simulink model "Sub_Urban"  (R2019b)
settings: Solver=FixedStepAuto  StartTime=0.0  StopTime=3600*24  FixedStep=Tstep  MaxStep=1800  RelTol=1e-3
InitFcn:
  | load('network_parameters')
  | Vnom=400/sqrt(3);
  | Tstep=30*60;
  | MV_LV_transf=0;
StopFcn:
  | run('Simulink_Data.m')
undefined symbols (not defined in the file or in its folder): C_xlpe_185_90, D11, Delta, L_2x16mm, L_2x22mm, L_4x100mm, L_4x16mm, L_4x22mm, L_4x50mm, L_xlpe_185_90, LC, Line_length, R_2x16mm, R_2x22mm, R_4x100mm, R_4x16mm, R_4x22mm, R_4x50mm, R_xlpe_185_90, Source_Voltage
libraries: myLibrary x125, powerlib x89
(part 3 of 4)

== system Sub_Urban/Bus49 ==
  Three Phase Zero Bus : myLibrary/Three Phase Zero Bus  SystemSampleTime=-1  Latency=0  AutoFrameSizeCalculation=off
  To Workspace I : ToWorkspace  VariableName=I49  SaveFormat=Structure With Time  SampleTime=-1
  To Workspace V : ToWorkspace  VariableName=Bus49  SaveFormat=Structure With Time  SampleTime=-1
  A : PMIOPort  Tag=PMCPort  Side=Left
  B : PMIOPort  Tag=PMCPort  Port=2  Side=Left
  C : PMIOPort  Tag=PMCPort  Port=3  Side=Left
  N : PMIOPort  Tag=PMCPort  Port=4  Side=Left
  a : PMIOPort  Tag=PMCPort  Port=5  Side=Right
  b : PMIOPort  Tag=PMCPort  Port=6  Side=Right
  c : PMIOPort  Tag=PMCPort  Port=7  Side=Right
  n : PMIOPort  Tag=PMCPort  Port=8  Side=Right
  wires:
  Three Phase Zero Bus/1 -> To Workspace V/1
  Three Phase Zero Bus/2 -> To Workspace I/1
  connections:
  A/RConn1 -- Three Phase Zero Bus/LConn1
  B/RConn1 -- Three Phase Zero Bus/LConn2
  C/RConn1 -- Three Phase Zero Bus/LConn3
  N/RConn1 -- Three Phase Zero Bus/LConn4
  a/RConn1 -- Three Phase Zero Bus/RConn1
  b/RConn1 -- Three Phase Zero Bus/RConn2
  c/RConn1 -- Three Phase Zero Bus/RConn3
  n/RConn1 -- Three Phase Zero Bus/RConn4

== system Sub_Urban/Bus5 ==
  Three Phase Zero Bus : myLibrary/Three Phase Zero Bus  SystemSampleTime=-1  Latency=0  AutoFrameSizeCalculation=off
  To Workspace I : ToWorkspace  VariableName=I5  SaveFormat=Structure With Time  SampleTime=-1
  To Workspace V : ToWorkspace  VariableName=Bus5  SaveFormat=Structure With Time  SampleTime=-1
  A : PMIOPort  Tag=PMCPort  Side=Left
  B : PMIOPort  Tag=PMCPort  Port=2  Side=Left
  C : PMIOPort  Tag=PMCPort  Port=3  Side=Left
  N : PMIOPort  Tag=PMCPort  Port=4  Side=Left
  a : PMIOPort  Tag=PMCPort  Port=5  Side=Right
  b : PMIOPort  Tag=PMCPort  Port=6  Side=Right
  c : PMIOPort  Tag=PMCPort  Port=7  Side=Right
  n : PMIOPort  Tag=PMCPort  Port=8  Side=Right
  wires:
  Three Phase Zero Bus/1 -> To Workspace V/1
  Three Phase Zero Bus/2 -> To Workspace I/1
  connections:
  A/RConn1 -- Three Phase Zero Bus/LConn1
  B/RConn1 -- Three Phase Zero Bus/LConn2
  C/RConn1 -- Three Phase Zero Bus/LConn3
  N/RConn1 -- Three Phase Zero Bus/LConn4
  a/RConn1 -- Three Phase Zero Bus/RConn1
  b/RConn1 -- Three Phase Zero Bus/RConn2
  c/RConn1 -- Three Phase Zero Bus/RConn3
  n/RConn1 -- Three Phase Zero Bus/RConn4

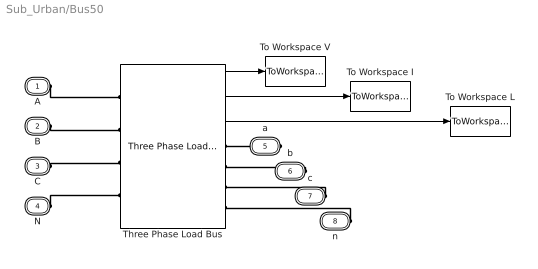
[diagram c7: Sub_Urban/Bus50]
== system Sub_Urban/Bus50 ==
  Three Phase Load Bus : myLibrary/Three Phase Load Bus  SystemSampleTime=-1  Latency=0  AutoFrameSizeCalculation=off
  To Workspace I : ToWorkspace  VariableName=I50  SaveFormat=Structure With Time  SampleTime=-1
  To Workspace L : ToWorkspace  VariableName=Load32  SaveFormat=Structure With Time  SampleTime=-1
  To Workspace V : ToWorkspace  VariableName=Bus50  SaveFormat=Structure With Time  SampleTime=-1
  A : PMIOPort  Tag=PMCPort  Side=Left
  B : PMIOPort  Tag=PMCPort  Port=2  Side=Left
  C : PMIOPort  Tag=PMCPort  Port=3  Side=Left
  N : PMIOPort  Tag=PMCPort  Port=4  Side=Left
  a : PMIOPort  Tag=PMCPort  Port=5  Side=Right
  b : PMIOPort  Tag=PMCPort  Port=6  Side=Right
  c : PMIOPort  Tag=PMCPort  Port=7  Side=Right
  n : PMIOPort  Tag=PMCPort  Port=8  Side=Right
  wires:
  Three Phase Load Bus/1 -> To Workspace V/1
  Three Phase Load Bus/2 -> To Workspace I/1
  Three Phase Load Bus/3 -> To Workspace L/1
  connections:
  N/RConn1 -- Three Phase Load Bus/LConn4
  C/RConn1 -- Three Phase Load Bus/LConn3
  n/RConn1 -- Three Phase Load Bus/RConn4
  B/RConn1 -- Three Phase Load Bus/LConn2
  A/RConn1 -- Three Phase Load Bus/LConn1
  b/RConn1 -- Three Phase Load Bus/RConn2
  c/RConn1 -- Three Phase Load Bus/RConn3
  a/RConn1 -- Three Phase Load Bus/RConn1

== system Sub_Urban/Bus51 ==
  Constant : Constant  Value=Ph
  Single Phase Load Bus : myLibrary/Single Phase Load Bus  SystemSampleTime=-1  Latency=0  AutoFrameSizeCalculation=off
  To Workspace I : ToWorkspace  VariableName=I51  SaveFormat=Structure With Time  SampleTime=-1
  To Workspace L : ToWorkspace  VariableName=Load33  SaveFormat=Structure With Time  SampleTime=-1
  To Workspace V : ToWorkspace  VariableName=Bus51  SaveFormat=Structure With Time  SampleTime=-1
  Phase : PMIOPort  Tag=PMCPort  Side=Left
  N : PMIOPort  Tag=PMCPort  Port=2  Side=Left
  phase : PMIOPort  Tag=PMCPort  Port=3  Side=Right
  n : PMIOPort  Tag=PMCPort  Port=4  Side=Right
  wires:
  Constant/1 -> Single Phase Load Bus/1
  Single Phase Load Bus/1 -> To Workspace V/1
  Single Phase Load Bus/2 -> To Workspace I/1
  Single Phase Load Bus/3 -> To Workspace L/1
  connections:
  Phase/RConn1 -- Single Phase Load Bus/LConn1
  N/RConn1 -- Single Phase Load Bus/LConn2
  phase/RConn1 -- Single Phase Load Bus/RConn1
  n/RConn1 -- Single Phase Load Bus/RConn2

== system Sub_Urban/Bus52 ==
  Three Phase Zero Bus : myLibrary/Three Phase Zero Bus  SystemSampleTime=-1  Latency=0  AutoFrameSizeCalculation=off
  To Workspace I : ToWorkspace  VariableName=I52  SaveFormat=Structure With Time  SampleTime=-1
  To Workspace V : ToWorkspace  VariableName=Bus52  SaveFormat=Structure With Time  SampleTime=-1
  A : PMIOPort  Tag=PMCPort  Side=Left
  B : PMIOPort  Tag=PMCPort  Port=2  Side=Left
  C : PMIOPort  Tag=PMCPort  Port=3  Side=Left
  N : PMIOPort  Tag=PMCPort  Port=4  Side=Left
  a : PMIOPort  Tag=PMCPort  Port=5  Side=Right
  b : PMIOPort  Tag=PMCPort  Port=6  Side=Right
  c : PMIOPort  Tag=PMCPort  Port=7  Side=Right
  n : PMIOPort  Tag=PMCPort  Port=8  Side=Right
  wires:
  Three Phase Zero Bus/1 -> To Workspace V/1
  Three Phase Zero Bus/2 -> To Workspace I/1
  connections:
  A/RConn1 -- Three Phase Zero Bus/LConn1
  B/RConn1 -- Three Phase Zero Bus/LConn2
  C/RConn1 -- Three Phase Zero Bus/LConn3
  N/RConn1 -- Three Phase Zero Bus/LConn4
  a/RConn1 -- Three Phase Zero Bus/RConn1
  b/RConn1 -- Three Phase Zero Bus/RConn2
  c/RConn1 -- Three Phase Zero Bus/RConn3
  n/RConn1 -- Three Phase Zero Bus/RConn4

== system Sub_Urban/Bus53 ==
  Constant : Constant  Value=Ph
  Single Phase Load Bus : myLibrary/Single Phase Load Bus  SystemSampleTime=-1  Latency=0  AutoFrameSizeCalculation=off
  To Workspace I : ToWorkspace  VariableName=I53  SaveFormat=Structure With Time  SampleTime=-1
  To Workspace L : ToWorkspace  VariableName=Load34  SaveFormat=Structure With Time  SampleTime=-1
  To Workspace V : ToWorkspace  VariableName=Bus53  SaveFormat=Structure With Time  SampleTime=-1
  Phase : PMIOPort  Tag=PMCPort  Side=Left
  N : PMIOPort  Tag=PMCPort  Port=2  Side=Left
  phase : PMIOPort  Tag=PMCPort  Port=3  Side=Right
  n : PMIOPort  Tag=PMCPort  Port=4  Side=Right
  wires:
  Constant/1 -> Single Phase Load Bus/1
  Single Phase Load Bus/1 -> To Workspace V/1
  Single Phase Load Bus/2 -> To Workspace I/1
  Single Phase Load Bus/3 -> To Workspace L/1
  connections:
  Phase/RConn1 -- Single Phase Load Bus/LConn1
  N/RConn1 -- Single Phase Load Bus/LConn2
  phase/RConn1 -- Single Phase Load Bus/RConn1
  n/RConn1 -- Single Phase Load Bus/RConn2

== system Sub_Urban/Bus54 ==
  Constant : Constant  Value=Ph
  Single Phase Load Bus : myLibrary/Single Phase Load Bus  SystemSampleTime=-1  Latency=0  AutoFrameSizeCalculation=off
  To Workspace I : ToWorkspace  VariableName=I54  SaveFormat=Structure With Time  SampleTime=-1
  To Workspace L : ToWorkspace  VariableName=Load35  SaveFormat=Structure With Time  SampleTime=-1
  To Workspace V : ToWorkspace  VariableName=Bus54  SaveFormat=Structure With Time  SampleTime=-1
  Phase : PMIOPort  Tag=PMCPort  Side=Left
  N : PMIOPort  Tag=PMCPort  Port=2  Side=Left
  phase : PMIOPort  Tag=PMCPort  Port=3  Side=Right
  n : PMIOPort  Tag=PMCPort  Port=4  Side=Right
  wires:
  Constant/1 -> Single Phase Load Bus/1
  Single Phase Load Bus/1 -> To Workspace V/1
  Single Phase Load Bus/2 -> To Workspace I/1
  Single Phase Load Bus/3 -> To Workspace L/1
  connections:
  Phase/RConn1 -- Single Phase Load Bus/LConn1
  N/RConn1 -- Single Phase Load Bus/LConn2
  phase/RConn1 -- Single Phase Load Bus/RConn1
  n/RConn1 -- Single Phase Load Bus/RConn2

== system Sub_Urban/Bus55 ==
  Three Phase Zero Bus : myLibrary/Three Phase Zero Bus  SystemSampleTime=-1  Latency=0  AutoFrameSizeCalculation=off
  To Workspace I : ToWorkspace  VariableName=I55  SaveFormat=Structure With Time  SampleTime=-1
  To Workspace V : ToWorkspace  VariableName=Bus55  SaveFormat=Structure With Time  SampleTime=-1
  A : PMIOPort  Tag=PMCPort  Side=Left
  B : PMIOPort  Tag=PMCPort  Port=2  Side=Left
  C : PMIOPort  Tag=PMCPort  Port=3  Side=Left
  N : PMIOPort  Tag=PMCPort  Port=4  Side=Left
  a : PMIOPort  Tag=PMCPort  Port=5  Side=Right
  b : PMIOPort  Tag=PMCPort  Port=6  Side=Right
  c : PMIOPort  Tag=PMCPort  Port=7  Side=Right
  n : PMIOPort  Tag=PMCPort  Port=8  Side=Right
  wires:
  Three Phase Zero Bus/1 -> To Workspace V/1
  Three Phase Zero Bus/2 -> To Workspace I/1
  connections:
  A/RConn1 -- Three Phase Zero Bus/LConn1
  B/RConn1 -- Three Phase Zero Bus/LConn2
  C/RConn1 -- Three Phase Zero Bus/LConn3
  N/RConn1 -- Three Phase Zero Bus/LConn4
  a/RConn1 -- Three Phase Zero Bus/RConn1
  b/RConn1 -- Three Phase Zero Bus/RConn2
  c/RConn1 -- Three Phase Zero Bus/RConn3
  n/RConn1 -- Three Phase Zero Bus/RConn4

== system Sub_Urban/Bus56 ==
  Constant : Constant  Value=Ph
  Single Phase Load Bus : myLibrary/Single Phase Load Bus  SystemSampleTime=-1  Latency=0  AutoFrameSizeCalculation=off
  To Workspace I : ToWorkspace  VariableName=I56  SaveFormat=Structure With Time  SampleTime=-1
  To Workspace L : ToWorkspace  VariableName=Load36  SaveFormat=Structure With Time  SampleTime=-1
  To Workspace V : ToWorkspace  VariableName=Bus56  SaveFormat=Structure With Time  SampleTime=-1
  Phase : PMIOPort  Tag=PMCPort  Side=Left
  N : PMIOPort  Tag=PMCPort  Port=2  Side=Left
  phase : PMIOPort  Tag=PMCPort  Port=3  Side=Right
  n : PMIOPort  Tag=PMCPort  Port=4  Side=Right
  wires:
  Constant/1 -> Single Phase Load Bus/1
  Single Phase Load Bus/1 -> To Workspace V/1
  Single Phase Load Bus/2 -> To Workspace I/1
  Single Phase Load Bus/3 -> To Workspace L/1
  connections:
  Phase/RConn1 -- Single Phase Load Bus/LConn1
  N/RConn1 -- Single Phase Load Bus/LConn2
  phase/RConn1 -- Single Phase Load Bus/RConn1
  n/RConn1 -- Single Phase Load Bus/RConn2

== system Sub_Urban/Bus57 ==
  Constant : Constant  Value=Ph
  Single Phase Load Bus : myLibrary/Single Phase Load Bus  SystemSampleTime=-1  Latency=0  AutoFrameSizeCalculation=off
  To Workspace I : ToWorkspace  VariableName=I57  SaveFormat=Structure With Time  SampleTime=-1
  To Workspace L : ToWorkspace  VariableName=Load37  SaveFormat=Structure With Time  SampleTime=-1
  To Workspace V : ToWorkspace  VariableName=Bus57  SaveFormat=Structure With Time  SampleTime=-1
  Phase : PMIOPort  Tag=PMCPort  Side=Left
  N : PMIOPort  Tag=PMCPort  Port=2  Side=Left
  phase : PMIOPort  Tag=PMCPort  Port=3  Side=Right
  n : PMIOPort  Tag=PMCPort  Port=4  Side=Right
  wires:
  Constant/1 -> Single Phase Load Bus/1
  Single Phase Load Bus/1 -> To Workspace V/1
  Single Phase Load Bus/2 -> To Workspace I/1
  Single Phase Load Bus/3 -> To Workspace L/1
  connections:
  Phase/RConn1 -- Single Phase Load Bus/LConn1
  N/RConn1 -- Single Phase Load Bus/LConn2
  phase/RConn1 -- Single Phase Load Bus/RConn1
  n/RConn1 -- Single Phase Load Bus/RConn2

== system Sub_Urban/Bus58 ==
  Three Phase Zero Bus : myLibrary/Three Phase Zero Bus  SystemSampleTime=-1  Latency=0  AutoFrameSizeCalculation=off
  To Workspace I : ToWorkspace  VariableName=I58  SaveFormat=Structure With Time  SampleTime=-1
  To Workspace V : ToWorkspace  VariableName=Bus58  SaveFormat=Structure With Time  SampleTime=-1
  A : PMIOPort  Tag=PMCPort  Side=Left
  B : PMIOPort  Tag=PMCPort  Port=2  Side=Left
  C : PMIOPort  Tag=PMCPort  Port=3  Side=Left
  N : PMIOPort  Tag=PMCPort  Port=4  Side=Left
  a : PMIOPort  Tag=PMCPort  Port=5  Side=Right
  b : PMIOPort  Tag=PMCPort  Port=6  Side=Right
  c : PMIOPort  Tag=PMCPort  Port=7  Side=Right
  n : PMIOPort  Tag=PMCPort  Port=8  Side=Right
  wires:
  Three Phase Zero Bus/1 -> To Workspace V/1
  Three Phase Zero Bus/2 -> To Workspace I/1
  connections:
  A/RConn1 -- Three Phase Zero Bus/LConn1
  B/RConn1 -- Three Phase Zero Bus/LConn2
  C/RConn1 -- Three Phase Zero Bus/LConn3
  N/RConn1 -- Three Phase Zero Bus/LConn4
  a/RConn1 -- Three Phase Zero Bus/RConn1
  b/RConn1 -- Three Phase Zero Bus/RConn2
  c/RConn1 -- Three Phase Zero Bus/RConn3
  n/RConn1 -- Three Phase Zero Bus/RConn4

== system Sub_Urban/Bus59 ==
  Constant : Constant  Value=Ph
  Single Phase Load Bus : myLibrary/Single Phase Load Bus  SystemSampleTime=-1  Latency=0  AutoFrameSizeCalculation=off
  To Workspace I : ToWorkspace  VariableName=I59  SaveFormat=Structure With Time  SampleTime=-1
  To Workspace L : ToWorkspace  VariableName=Load38  SaveFormat=Structure With Time  SampleTime=-1
  To Workspace V : ToWorkspace  VariableName=Bus59  SaveFormat=Structure With Time  SampleTime=-1
  Phase : PMIOPort  Tag=PMCPort  Side=Left
  N : PMIOPort  Tag=PMCPort  Port=2  Side=Left
  phase : PMIOPort  Tag=PMCPort  Port=3  Side=Right
  n : PMIOPort  Tag=PMCPort  Port=4  Side=Right
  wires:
  Constant/1 -> Single Phase Load Bus/1
  Single Phase Load Bus/1 -> To Workspace V/1
  Single Phase Load Bus/2 -> To Workspace I/1
  Single Phase Load Bus/3 -> To Workspace L/1
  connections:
  Phase/RConn1 -- Single Phase Load Bus/LConn1
  N/RConn1 -- Single Phase Load Bus/LConn2
  phase/RConn1 -- Single Phase Load Bus/RConn1
  n/RConn1 -- Single Phase Load Bus/RConn2

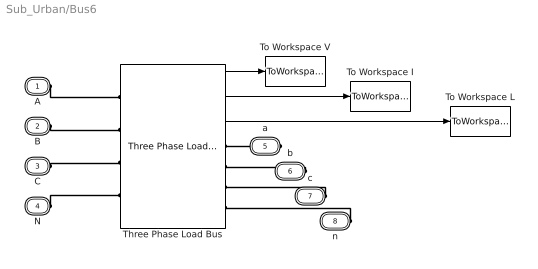
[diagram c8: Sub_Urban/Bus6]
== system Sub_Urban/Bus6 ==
  Three Phase Load Bus : myLibrary/Three Phase Load Bus  SystemSampleTime=-1  Latency=0  AutoFrameSizeCalculation=off
  To Workspace I : ToWorkspace  VariableName=I6  SaveFormat=Structure With Time  SampleTime=-1
  To Workspace L : ToWorkspace  VariableName=Load2  SaveFormat=Structure With Time  SampleTime=-1
  To Workspace V : ToWorkspace  VariableName=Bus6  SaveFormat=Structure With Time  SampleTime=-1
  A : PMIOPort  Tag=PMCPort  Side=Left
  B : PMIOPort  Tag=PMCPort  Port=2  Side=Left
  C : PMIOPort  Tag=PMCPort  Port=3  Side=Left
  N : PMIOPort  Tag=PMCPort  Port=4  Side=Left
  a : PMIOPort  Tag=PMCPort  Port=5  Side=Right
  b : PMIOPort  Tag=PMCPort  Port=6  Side=Right
  c : PMIOPort  Tag=PMCPort  Port=7  Side=Right
  n : PMIOPort  Tag=PMCPort  Port=8  Side=Right
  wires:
  Three Phase Load Bus/1 -> To Workspace V/1
  Three Phase Load Bus/2 -> To Workspace I/1
  Three Phase Load Bus/3 -> To Workspace L/1
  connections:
  N/RConn1 -- Three Phase Load Bus/LConn4
  C/RConn1 -- Three Phase Load Bus/LConn3
  n/RConn1 -- Three Phase Load Bus/RConn4
  B/RConn1 -- Three Phase Load Bus/LConn2
  A/RConn1 -- Three Phase Load Bus/LConn1
  b/RConn1 -- Three Phase Load Bus/RConn2
  c/RConn1 -- Three Phase Load Bus/RConn3
  a/RConn1 -- Three Phase Load Bus/RConn1

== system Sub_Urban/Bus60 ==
  Constant : Constant  Value=Ph
  Single Phase Load Bus : myLibrary/Single Phase Load Bus  SystemSampleTime=-1  Latency=0  AutoFrameSizeCalculation=off
  To Workspace I : ToWorkspace  VariableName=I60  SaveFormat=Structure With Time  SampleTime=-1
  To Workspace L : ToWorkspace  VariableName=Load39  SaveFormat=Structure With Time  SampleTime=-1
  To Workspace V : ToWorkspace  VariableName=Bus60  SaveFormat=Structure With Time  SampleTime=-1
  Phase : PMIOPort  Tag=PMCPort  Side=Left
  N : PMIOPort  Tag=PMCPort  Port=2  Side=Left
  phase : PMIOPort  Tag=PMCPort  Port=3  Side=Right
  n : PMIOPort  Tag=PMCPort  Port=4  Side=Right
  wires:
  Constant/1 -> Single Phase Load Bus/1
  Single Phase Load Bus/1 -> To Workspace V/1
  Single Phase Load Bus/2 -> To Workspace I/1
  Single Phase Load Bus/3 -> To Workspace L/1
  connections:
  Phase/RConn1 -- Single Phase Load Bus/LConn1
  N/RConn1 -- Single Phase Load Bus/LConn2
  phase/RConn1 -- Single Phase Load Bus/RConn1
  n/RConn1 -- Single Phase Load Bus/RConn2

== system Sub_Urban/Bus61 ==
  Constant : Constant  Value=Ph
  Single Phase Load Bus : myLibrary/Single Phase Load Bus  SystemSampleTime=-1  Latency=0  AutoFrameSizeCalculation=off
  To Workspace I : ToWorkspace  VariableName=I61  SaveFormat=Structure With Time  SampleTime=-1
  To Workspace L : ToWorkspace  VariableName=Load40  SaveFormat=Structure With Time  SampleTime=-1
  To Workspace V : ToWorkspace  VariableName=Bus61  SaveFormat=Structure With Time  SampleTime=-1
  Phase : PMIOPort  Tag=PMCPort  Side=Left
  N : PMIOPort  Tag=PMCPort  Port=2  Side=Left
  phase : PMIOPort  Tag=PMCPort  Port=3  Side=Right
  n : PMIOPort  Tag=PMCPort  Port=4  Side=Right
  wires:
  Constant/1 -> Single Phase Load Bus/1
  Single Phase Load Bus/1 -> To Workspace V/1
  Single Phase Load Bus/2 -> To Workspace I/1
  Single Phase Load Bus/3 -> To Workspace L/1
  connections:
  Phase/RConn1 -- Single Phase Load Bus/LConn1
  N/RConn1 -- Single Phase Load Bus/LConn2
  phase/RConn1 -- Single Phase Load Bus/RConn1
  n/RConn1 -- Single Phase Load Bus/RConn2

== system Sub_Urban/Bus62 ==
  Three Phase Zero Bus : myLibrary/Three Phase Zero Bus  SystemSampleTime=-1  Latency=0  AutoFrameSizeCalculation=off
  To Workspace I : ToWorkspace  VariableName=I62  SaveFormat=Structure With Time  SampleTime=-1
  To Workspace V : ToWorkspace  VariableName=Bus62  SaveFormat=Structure With Time  SampleTime=-1
  A : PMIOPort  Tag=PMCPort  Side=Left
  B : PMIOPort  Tag=PMCPort  Port=2  Side=Left
  C : PMIOPort  Tag=PMCPort  Port=3  Side=Left
  N : PMIOPort  Tag=PMCPort  Port=4  Side=Left
  a : PMIOPort  Tag=PMCPort  Port=5  Side=Right
  b : PMIOPort  Tag=PMCPort  Port=6  Side=Right
  c : PMIOPort  Tag=PMCPort  Port=7  Side=Right
  n : PMIOPort  Tag=PMCPort  Port=8  Side=Right
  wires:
  Three Phase Zero Bus/1 -> To Workspace V/1
  Three Phase Zero Bus/2 -> To Workspace I/1
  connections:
  A/RConn1 -- Three Phase Zero Bus/LConn1
  B/RConn1 -- Three Phase Zero Bus/LConn2
  C/RConn1 -- Three Phase Zero Bus/LConn3
  N/RConn1 -- Three Phase Zero Bus/LConn4
  a/RConn1 -- Three Phase Zero Bus/RConn1
  b/RConn1 -- Three Phase Zero Bus/RConn2
  c/RConn1 -- Three Phase Zero Bus/RConn3
  n/RConn1 -- Three Phase Zero Bus/RConn4

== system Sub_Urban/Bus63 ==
  Three Phase Zero Bus : myLibrary/Three Phase Zero Bus  SystemSampleTime=-1  Latency=0  AutoFrameSizeCalculation=off
  To Workspace I : ToWorkspace  VariableName=I63  SaveFormat=Structure With Time  SampleTime=-1
  To Workspace V : ToWorkspace  VariableName=Bus63  SaveFormat=Structure With Time  SampleTime=-1
  A : PMIOPort  Tag=PMCPort  Side=Left
  B : PMIOPort  Tag=PMCPort  Port=2  Side=Left
  C : PMIOPort  Tag=PMCPort  Port=3  Side=Left
  N : PMIOPort  Tag=PMCPort  Port=4  Side=Left
  a : PMIOPort  Tag=PMCPort  Port=5  Side=Right
  b : PMIOPort  Tag=PMCPort  Port=6  Side=Right
  c : PMIOPort  Tag=PMCPort  Port=7  Side=Right
  n : PMIOPort  Tag=PMCPort  Port=8  Side=Right
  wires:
  Three Phase Zero Bus/1 -> To Workspace V/1
  Three Phase Zero Bus/2 -> To Workspace I/1
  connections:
  A/RConn1 -- Three Phase Zero Bus/LConn1
  B/RConn1 -- Three Phase Zero Bus/LConn2
  C/RConn1 -- Three Phase Zero Bus/LConn3
  N/RConn1 -- Three Phase Zero Bus/LConn4
  a/RConn1 -- Three Phase Zero Bus/RConn1
  b/RConn1 -- Three Phase Zero Bus/RConn2
  c/RConn1 -- Three Phase Zero Bus/RConn3
  n/RConn1 -- Three Phase Zero Bus/RConn4

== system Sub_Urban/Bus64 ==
  Three Phase Load Bus : myLibrary/Three Phase Load Bus  SystemSampleTime=-1  Latency=0  AutoFrameSizeCalculation=off
  To Workspace I : ToWorkspace  VariableName=I64  SaveFormat=Structure With Time  SampleTime=-1
  To Workspace L : ToWorkspace  VariableName=Load41  SaveFormat=Structure With Time  SampleTime=-1
  To Workspace V : ToWorkspace  VariableName=Bus64  SaveFormat=Structure With Time  SampleTime=-1
  A : PMIOPort  Tag=PMCPort  Side=Left
  B : PMIOPort  Tag=PMCPort  Port=2  Side=Left
  C : PMIOPort  Tag=PMCPort  Port=3  Side=Left
  N : PMIOPort  Tag=PMCPort  Port=4  Side=Left
  a : PMIOPort  Tag=PMCPort  Port=5  Side=Right
  b : PMIOPort  Tag=PMCPort  Port=6  Side=Right
  c : PMIOPort  Tag=PMCPort  Port=7  Side=Right
  n : PMIOPort  Tag=PMCPort  Port=8  Side=Right
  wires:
  Three Phase Load Bus/1 -> To Workspace V/1
  Three Phase Load Bus/2 -> To Workspace I/1
  Three Phase Load Bus/3 -> To Workspace L/1
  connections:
  N/RConn1 -- Three Phase Load Bus/LConn4
  C/RConn1 -- Three Phase Load Bus/LConn3
  n/RConn1 -- Three Phase Load Bus/RConn4
  B/RConn1 -- Three Phase Load Bus/LConn2
  A/RConn1 -- Three Phase Load Bus/LConn1
  b/RConn1 -- Three Phase Load Bus/RConn2
  c/RConn1 -- Three Phase Load Bus/RConn3
  a/RConn1 -- Three Phase Load Bus/RConn1

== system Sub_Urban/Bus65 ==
  Constant : Constant  Value=Ph
  Single Phase Load Bus : myLibrary/Single Phase Load Bus  SystemSampleTime=-1  Latency=0  AutoFrameSizeCalculation=off
  To Workspace I : ToWorkspace  VariableName=I65  SaveFormat=Structure With Time  SampleTime=-1
  To Workspace L : ToWorkspace  VariableName=Load42  SaveFormat=Structure With Time  SampleTime=-1
  To Workspace V : ToWorkspace  VariableName=Bus65  SaveFormat=Structure With Time  SampleTime=-1
  Phase : PMIOPort  Tag=PMCPort  Side=Left
  N : PMIOPort  Tag=PMCPort  Port=2  Side=Left
  phase : PMIOPort  Tag=PMCPort  Port=3  Side=Right
  n : PMIOPort  Tag=PMCPort  Port=4  Side=Right
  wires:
  Constant/1 -> Single Phase Load Bus/1
  Single Phase Load Bus/1 -> To Workspace V/1
  Single Phase Load Bus/2 -> To Workspace I/1
  Single Phase Load Bus/3 -> To Workspace L/1
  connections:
  Phase/RConn1 -- Single Phase Load Bus/LConn1
  N/RConn1 -- Single Phase Load Bus/LConn2
  phase/RConn1 -- Single Phase Load Bus/RConn1
  n/RConn1 -- Single Phase Load Bus/RConn2

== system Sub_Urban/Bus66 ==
  Three Phase Zero Bus : myLibrary/Three Phase Zero Bus  SystemSampleTime=-1  Latency=0  AutoFrameSizeCalculation=off
  To Workspace I : ToWorkspace  VariableName=I66  SaveFormat=Structure With Time  SampleTime=-1
  To Workspace V : ToWorkspace  VariableName=Bus66  SaveFormat=Structure With Time  SampleTime=-1
  A : PMIOPort  Tag=PMCPort  Side=Left
  B : PMIOPort  Tag=PMCPort  Port=2  Side=Left
  C : PMIOPort  Tag=PMCPort  Port=3  Side=Left
  N : PMIOPort  Tag=PMCPort  Port=4  Side=Left
  a : PMIOPort  Tag=PMCPort  Port=5  Side=Right
  b : PMIOPort  Tag=PMCPort  Port=6  Side=Right
  c : PMIOPort  Tag=PMCPort  Port=7  Side=Right
  n : PMIOPort  Tag=PMCPort  Port=8  Side=Right
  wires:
  Three Phase Zero Bus/1 -> To Workspace V/1
  Three Phase Zero Bus/2 -> To Workspace I/1
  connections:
  A/RConn1 -- Three Phase Zero Bus/LConn1
  B/RConn1 -- Three Phase Zero Bus/LConn2
  C/RConn1 -- Three Phase Zero Bus/LConn3
  N/RConn1 -- Three Phase Zero Bus/LConn4
  a/RConn1 -- Three Phase Zero Bus/RConn1
  b/RConn1 -- Three Phase Zero Bus/RConn2
  c/RConn1 -- Three Phase Zero Bus/RConn3
  n/RConn1 -- Three Phase Zero Bus/RConn4

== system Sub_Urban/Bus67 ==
  Constant : Constant  Value=Ph
  Single Phase Load Bus : myLibrary/Single Phase Load Bus  SystemSampleTime=-1  Latency=0  AutoFrameSizeCalculation=off
  To Workspace I : ToWorkspace  VariableName=I67  SaveFormat=Structure With Time  SampleTime=-1
  To Workspace L : ToWorkspace  VariableName=Load43  SaveFormat=Structure With Time  SampleTime=-1
  To Workspace V : ToWorkspace  VariableName=Bus67  SaveFormat=Structure With Time  SampleTime=-1
  Phase : PMIOPort  Tag=PMCPort  Side=Left
  N : PMIOPort  Tag=PMCPort  Port=2  Side=Left
  phase : PMIOPort  Tag=PMCPort  Port=3  Side=Right
  n : PMIOPort  Tag=PMCPort  Port=4  Side=Right
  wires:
  Constant/1 -> Single Phase Load Bus/1
  Single Phase Load Bus/1 -> To Workspace V/1
  Single Phase Load Bus/2 -> To Workspace I/1
  Single Phase Load Bus/3 -> To Workspace L/1
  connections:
  Phase/RConn1 -- Single Phase Load Bus/LConn1
  N/RConn1 -- Single Phase Load Bus/LConn2
  phase/RConn1 -- Single Phase Load Bus/RConn1
  n/RConn1 -- Single Phase Load Bus/RConn2

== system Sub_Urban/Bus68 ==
  Constant : Constant  Value=Ph
  Single Phase Load Bus : myLibrary/Single Phase Load Bus  SystemSampleTime=-1  Latency=0  AutoFrameSizeCalculation=off
  To Workspace I : ToWorkspace  VariableName=I68  SaveFormat=Structure With Time  SampleTime=-1
  To Workspace L : ToWorkspace  VariableName=Load44  SaveFormat=Structure With Time  SampleTime=-1
  To Workspace V : ToWorkspace  VariableName=Bus68  SaveFormat=Structure With Time  SampleTime=-1
  Phase : PMIOPort  Tag=PMCPort  Side=Left
  N : PMIOPort  Tag=PMCPort  Port=2  Side=Left
  phase : PMIOPort  Tag=PMCPort  Port=3  Side=Right
  n : PMIOPort  Tag=PMCPort  Port=4  Side=Right
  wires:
  Constant/1 -> Single Phase Load Bus/1
  Single Phase Load Bus/1 -> To Workspace V/1
  Single Phase Load Bus/2 -> To Workspace I/1
  Single Phase Load Bus/3 -> To Workspace L/1
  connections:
  Phase/RConn1 -- Single Phase Load Bus/LConn1
  N/RConn1 -- Single Phase Load Bus/LConn2
  phase/RConn1 -- Single Phase Load Bus/RConn1
  n/RConn1 -- Single Phase Load Bus/RConn2

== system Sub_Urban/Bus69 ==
  Constant : Constant  Value=Ph
  Single Phase Load Bus : myLibrary/Single Phase Load Bus  SystemSampleTime=-1  Latency=0  AutoFrameSizeCalculation=off
  To Workspace I : ToWorkspace  VariableName=I69  SaveFormat=Structure With Time  SampleTime=-1
  To Workspace L : ToWorkspace  VariableName=Load45  SaveFormat=Structure With Time  SampleTime=-1
  To Workspace V : ToWorkspace  VariableName=Bus69  SaveFormat=Structure With Time  SampleTime=-1
  Phase : PMIOPort  Tag=PMCPort  Side=Left
  N : PMIOPort  Tag=PMCPort  Port=2  Side=Left
  phase : PMIOPort  Tag=PMCPort  Port=3  Side=Right
  n : PMIOPort  Tag=PMCPort  Port=4  Side=Right
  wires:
  Constant/1 -> Single Phase Load Bus/1
  Single Phase Load Bus/1 -> To Workspace V/1
  Single Phase Load Bus/2 -> To Workspace I/1
  Single Phase Load Bus/3 -> To Workspace L/1
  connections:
  Phase/RConn1 -- Single Phase Load Bus/LConn1
  N/RConn1 -- Single Phase Load Bus/LConn2
  phase/RConn1 -- Single Phase Load Bus/RConn1
  n/RConn1 -- Single Phase Load Bus/RConn2

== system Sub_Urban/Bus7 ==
  Constant : Constant  Value=Ph
  Single Phase Load Bus : myLibrary/Single Phase Load Bus  SystemSampleTime=-1  Latency=0  AutoFrameSizeCalculation=off
  To Workspace I : ToWorkspace  VariableName=I7  SaveFormat=Structure With Time  SampleTime=-1
  To Workspace L : ToWorkspace  VariableName=Load3  SaveFormat=Structure With Time  SampleTime=-1
  To Workspace V : ToWorkspace  VariableName=Bus7  SaveFormat=Structure With Time  SampleTime=-1
  Phase : PMIOPort  Tag=PMCPort  Side=Left
  N : PMIOPort  Tag=PMCPort  Port=2  Side=Left
  phase : PMIOPort  Tag=PMCPort  Port=3  Side=Right
  n : PMIOPort  Tag=PMCPort  Port=4  Side=Right
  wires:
  Constant/1 -> Single Phase Load Bus/1
  Single Phase Load Bus/1 -> To Workspace V/1
  Single Phase Load Bus/2 -> To Workspace I/1
  Single Phase Load Bus/3 -> To Workspace L/1
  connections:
  Phase/RConn1 -- Single Phase Load Bus/LConn1
  N/RConn1 -- Single Phase Load Bus/LConn2
  phase/RConn1 -- Single Phase Load Bus/RConn1
  n/RConn1 -- Single Phase Load Bus/RConn2

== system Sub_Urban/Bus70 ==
  Three Phase Zero Bus : myLibrary/Three Phase Zero Bus  SystemSampleTime=-1  Latency=0  AutoFrameSizeCalculation=off
  To Workspace I : ToWorkspace  VariableName=I70  SaveFormat=Structure With Time  SampleTime=-1
  To Workspace V : ToWorkspace  VariableName=Bus70  SaveFormat=Structure With Time  SampleTime=-1
  A : PMIOPort  Tag=PMCPort  Side=Left
  B : PMIOPort  Tag=PMCPort  Port=2  Side=Left
  C : PMIOPort  Tag=PMCPort  Port=3  Side=Left
  N : PMIOPort  Tag=PMCPort  Port=4  Side=Left
  a : PMIOPort  Tag=PMCPort  Port=5  Side=Right
  b : PMIOPort  Tag=PMCPort  Port=6  Side=Right
  c : PMIOPort  Tag=PMCPort  Port=7  Side=Right
  n : PMIOPort  Tag=PMCPort  Port=8  Side=Right
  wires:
  Three Phase Zero Bus/1 -> To Workspace V/1
  Three Phase Zero Bus/2 -> To Workspace I/1
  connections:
  A/RConn1 -- Three Phase Zero Bus/LConn1
  B/RConn1 -- Three Phase Zero Bus/LConn2
  C/RConn1 -- Three Phase Zero Bus/LConn3
  N/RConn1 -- Three Phase Zero Bus/LConn4
  a/RConn1 -- Three Phase Zero Bus/RConn1
  b/RConn1 -- Three Phase Zero Bus/RConn2
  c/RConn1 -- Three Phase Zero Bus/RConn3
  n/RConn1 -- Three Phase Zero Bus/RConn4

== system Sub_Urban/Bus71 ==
  Constant : Constant  Value=Ph
  Single Phase Load Bus : myLibrary/Single Phase Load Bus  SystemSampleTime=-1  Latency=0  AutoFrameSizeCalculation=off
  To Workspace I : ToWorkspace  VariableName=I71  SaveFormat=Structure With Time  SampleTime=-1
  To Workspace L : ToWorkspace  VariableName=Load46  SaveFormat=Structure With Time  SampleTime=-1
  To Workspace V : ToWorkspace  VariableName=Bus71  SaveFormat=Structure With Time  SampleTime=-1
  Phase : PMIOPort  Tag=PMCPort  Side=Left
  N : PMIOPort  Tag=PMCPort  Port=2  Side=Left
  phase : PMIOPort  Tag=PMCPort  Port=3  Side=Right
  n : PMIOPort  Tag=PMCPort  Port=4  Side=Right
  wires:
  Constant/1 -> Single Phase Load Bus/1
  Single Phase Load Bus/1 -> To Workspace V/1
  Single Phase Load Bus/2 -> To Workspace I/1
  Single Phase Load Bus/3 -> To Workspace L/1
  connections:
  Phase/RConn1 -- Single Phase Load Bus/LConn1
  N/RConn1 -- Single Phase Load Bus/LConn2
  phase/RConn1 -- Single Phase Load Bus/RConn1
  n/RConn1 -- Single Phase Load Bus/RConn2

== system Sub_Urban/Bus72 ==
  Constant : Constant  Value=Ph
  Single Phase Load Bus : myLibrary/Single Phase Load Bus  SystemSampleTime=-1  Latency=0  AutoFrameSizeCalculation=off
  To Workspace I : ToWorkspace  VariableName=I72  SaveFormat=Structure With Time  SampleTime=-1
  To Workspace L : ToWorkspace  VariableName=Load47  SaveFormat=Structure With Time  SampleTime=-1
  To Workspace V : ToWorkspace  VariableName=Bus72  SaveFormat=Structure With Time  SampleTime=-1
  Phase : PMIOPort  Tag=PMCPort  Side=Left
  N : PMIOPort  Tag=PMCPort  Port=2  Side=Left
  phase : PMIOPort  Tag=PMCPort  Port=3  Side=Right
  n : PMIOPort  Tag=PMCPort  Port=4  Side=Right
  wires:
  Constant/1 -> Single Phase Load Bus/1
  Single Phase Load Bus/1 -> To Workspace V/1
  Single Phase Load Bus/2 -> To Workspace I/1
  Single Phase Load Bus/3 -> To Workspace L/1
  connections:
  Phase/RConn1 -- Single Phase Load Bus/LConn1
  N/RConn1 -- Single Phase Load Bus/LConn2
  phase/RConn1 -- Single Phase Load Bus/RConn1
  n/RConn1 -- Single Phase Load Bus/RConn2

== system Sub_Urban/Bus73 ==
  Constant : Constant  Value=Ph
  Single Phase Load Bus : myLibrary/Single Phase Load Bus  SystemSampleTime=-1  Latency=0  AutoFrameSizeCalculation=off
  To Workspace I : ToWorkspace  VariableName=I73  SaveFormat=Structure With Time  SampleTime=-1
  To Workspace L : ToWorkspace  VariableName=Load48  SaveFormat=Structure With Time  SampleTime=-1
  To Workspace V : ToWorkspace  VariableName=Bus73  SaveFormat=Structure With Time  SampleTime=-1
  Phase : PMIOPort  Tag=PMCPort  Side=Left
  N : PMIOPort  Tag=PMCPort  Port=2  Side=Left
  phase : PMIOPort  Tag=PMCPort  Port=3  Side=Right
  n : PMIOPort  Tag=PMCPort  Port=4  Side=Right
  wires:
  Constant/1 -> Single Phase Load Bus/1
  Single Phase Load Bus/1 -> To Workspace V/1
  Single Phase Load Bus/2 -> To Workspace I/1
  Single Phase Load Bus/3 -> To Workspace L/1
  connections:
  Phase/RConn1 -- Single Phase Load Bus/LConn1
  N/RConn1 -- Single Phase Load Bus/LConn2
  phase/RConn1 -- Single Phase Load Bus/RConn1
  n/RConn1 -- Single Phase Load Bus/RConn2

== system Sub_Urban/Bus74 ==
  Three Phase Load Bus : myLibrary/Three Phase Load Bus  SystemSampleTime=-1  Latency=0  AutoFrameSizeCalculation=off
  To Workspace I : ToWorkspace  VariableName=I74  SaveFormat=Structure With Time  SampleTime=-1
  To Workspace L : ToWorkspace  VariableName=Load49  SaveFormat=Structure With Time  SampleTime=-1
  To Workspace V : ToWorkspace  VariableName=Bus74  SaveFormat=Structure With Time  SampleTime=-1
  A : PMIOPort  Tag=PMCPort  Side=Left
  B : PMIOPort  Tag=PMCPort  Port=2  Side=Left
  C : PMIOPort  Tag=PMCPort  Port=3  Side=Left
  N : PMIOPort  Tag=PMCPort  Port=4  Side=Left
  a : PMIOPort  Tag=PMCPort  Port=5  Side=Right
  b : PMIOPort  Tag=PMCPort  Port=6  Side=Right
  c : PMIOPort  Tag=PMCPort  Port=7  Side=Right
  n : PMIOPort  Tag=PMCPort  Port=8  Side=Right
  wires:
  Three Phase Load Bus/1 -> To Workspace V/1
  Three Phase Load Bus/2 -> To Workspace I/1
  Three Phase Load Bus/3 -> To Workspace L/1
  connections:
  N/RConn1 -- Three Phase Load Bus/LConn4
  C/RConn1 -- Three Phase Load Bus/LConn3
  n/RConn1 -- Three Phase Load Bus/RConn4
  B/RConn1 -- Three Phase Load Bus/LConn2
  A/RConn1 -- Three Phase Load Bus/LConn1
  b/RConn1 -- Three Phase Load Bus/RConn2
  c/RConn1 -- Three Phase Load Bus/RConn3
  a/RConn1 -- Three Phase Load Bus/RConn1

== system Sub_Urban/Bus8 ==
  Constant : Constant  Value=Ph
  Single Phase Load Bus : myLibrary/Single Phase Load Bus  SystemSampleTime=-1  Latency=0  AutoFrameSizeCalculation=off
  To Workspace I : ToWorkspace  VariableName=I8  SaveFormat=Structure With Time  SampleTime=-1
  To Workspace L : ToWorkspace  VariableName=Load4  SaveFormat=Structure With Time  SampleTime=-1
  To Workspace V : ToWorkspace  VariableName=Bus8  SaveFormat=Structure With Time  SampleTime=-1
  Phase : PMIOPort  Tag=PMCPort  Side=Left
  N : PMIOPort  Tag=PMCPort  Port=2  Side=Left
  phase : PMIOPort  Tag=PMCPort  Port=3  Side=Right
  n : PMIOPort  Tag=PMCPort  Port=4  Side=Right
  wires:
  Constant/1 -> Single Phase Load Bus/1
  Single Phase Load Bus/1 -> To Workspace V/1
  Single Phase Load Bus/2 -> To Workspace I/1
  Single Phase Load Bus/3 -> To Workspace L/1
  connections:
  Phase/RConn1 -- Single Phase Load Bus/LConn1
  N/RConn1 -- Single Phase Load Bus/LConn2
  phase/RConn1 -- Single Phase Load Bus/RConn1
  n/RConn1 -- Single Phase Load Bus/RConn2

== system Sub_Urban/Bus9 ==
  Three Phase Zero Bus : myLibrary/Three Phase Zero Bus  SystemSampleTime=-1  Latency=0  AutoFrameSizeCalculation=off
  To Workspace I : ToWorkspace  VariableName=I9  SaveFormat=Structure With Time  SampleTime=-1
  To Workspace V : ToWorkspace  VariableName=Bus9  SaveFormat=Structure With Time  SampleTime=-1
  A : PMIOPort  Tag=PMCPort  Side=Left
  B : PMIOPort  Tag=PMCPort  Port=2  Side=Left
  C : PMIOPort  Tag=PMCPort  Port=3  Side=Left
  N : PMIOPort  Tag=PMCPort  Port=4  Side=Left
  a : PMIOPort  Tag=PMCPort  Port=5  Side=Right
  b : PMIOPort  Tag=PMCPort  Port=6  Side=Right
  c : PMIOPort  Tag=PMCPort  Port=7  Side=Right
  n : PMIOPort  Tag=PMCPort  Port=8  Side=Right
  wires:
  Three Phase Zero Bus/1 -> To Workspace V/1
  Three Phase Zero Bus/2 -> To Workspace I/1
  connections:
  A/RConn1 -- Three Phase Zero Bus/LConn1
  B/RConn1 -- Three Phase Zero Bus/LConn2
  C/RConn1 -- Three Phase Zero Bus/LConn3
  N/RConn1 -- Three Phase Zero Bus/LConn4
  a/RConn1 -- Three Phase Zero Bus/RConn1
  b/RConn1 -- Three Phase Zero Bus/RConn2
  c/RConn1 -- Three Phase Zero Bus/RConn3
  n/RConn1 -- Three Phase Zero Bus/RConn4

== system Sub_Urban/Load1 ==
  TPDL - Three-Phase Dynamic Load : myLibrary/TPDL - Three-Phase Dynamic Load  Load_Profile=LC(1)
  A : PMIOPort  Side=Left
  B : PMIOPort  Port=2  Side=Left
  C : PMIOPort  Port=3  Side=Left
  n : PMIOPort  Port=4  Side=Left
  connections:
  A/RConn1 -- TPDL - Three-Phase Dynamic Load/LConn1
  TPDL - Three-Phase Dynamic Load/LConn2 -- B/RConn1
  C/RConn1 -- TPDL - Three-Phase Dynamic Load/LConn3
  n/RConn1 -- TPDL - Three-Phase Dynamic Load/LConn4

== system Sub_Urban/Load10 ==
  SPDL - Single Phase Dynamic Load (Phasor) : myLibrary/SPDL - Single Phase Dynamic Load (Phasor)  Load_Profile=LC(10)  Phase=3
  Ph : PMIOPort  Side=Left
  n : PMIOPort  Port=2  Side=Left
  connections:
  Ph/RConn1 -- SPDL - Single Phase Dynamic Load (Phasor)/LConn1
  n/RConn1 -- SPDL - Single Phase Dynamic Load (Phasor)/LConn2

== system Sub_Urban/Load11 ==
  SPDL - Single Phase Dynamic Load (Phasor) : myLibrary/SPDL - Single Phase Dynamic Load (Phasor)  Load_Profile=LC(11)  Phase=3
  Ph : PMIOPort  Side=Left
  n : PMIOPort  Port=2  Side=Left
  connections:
  Ph/RConn1 -- SPDL - Single Phase Dynamic Load (Phasor)/LConn1
  n/RConn1 -- SPDL - Single Phase Dynamic Load (Phasor)/LConn2

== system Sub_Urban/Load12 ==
  SPDL - Single Phase Dynamic Load (Phasor) : myLibrary/SPDL - Single Phase Dynamic Load (Phasor)  Load_Profile=LC(12)  Phase=3
  Ph : PMIOPort  Side=Left
  n : PMIOPort  Port=2  Side=Left
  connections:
  Ph/RConn1 -- SPDL - Single Phase Dynamic Load (Phasor)/LConn1
  n/RConn1 -- SPDL - Single Phase Dynamic Load (Phasor)/LConn2

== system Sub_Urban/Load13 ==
  SPDL - Single Phase Dynamic Load (Phasor) : myLibrary/SPDL - Single Phase Dynamic Load (Phasor)  Load_Profile=LC(13)  Phase=3
  Ph : PMIOPort  Side=Left
  n : PMIOPort  Port=2  Side=Left
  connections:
  Ph/RConn1 -- SPDL - Single Phase Dynamic Load (Phasor)/LConn1
  n/RConn1 -- SPDL - Single Phase Dynamic Load (Phasor)/LConn2

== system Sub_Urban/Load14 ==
  SPDL - Single Phase Dynamic Load (Phasor) : myLibrary/SPDL - Single Phase Dynamic Load (Phasor)  Load_Profile=LC(14)  Phase=3
  Ph : PMIOPort  Side=Left
  n : PMIOPort  Port=2  Side=Left
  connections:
  Ph/RConn1 -- SPDL - Single Phase Dynamic Load (Phasor)/LConn1
  n/RConn1 -- SPDL - Single Phase Dynamic Load (Phasor)/LConn2

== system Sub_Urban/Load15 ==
  SPDL - Single Phase Dynamic Load (Phasor) : myLibrary/SPDL - Single Phase Dynamic Load (Phasor)  Load_Profile=LC(15)  Phase=1
  Ph : PMIOPort  Side=Left
  n : PMIOPort  Port=2  Side=Left
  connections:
  Ph/RConn1 -- SPDL - Single Phase Dynamic Load (Phasor)/LConn1
  n/RConn1 -- SPDL - Single Phase Dynamic Load (Phasor)/LConn2

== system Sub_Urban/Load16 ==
  TPDL - Three-Phase Dynamic Load : myLibrary/TPDL - Three-Phase Dynamic Load  Load_Profile=LC(16)
  A : PMIOPort  Side=Left
  B : PMIOPort  Port=2  Side=Left
  C : PMIOPort  Port=3  Side=Left
  n : PMIOPort  Port=4  Side=Left
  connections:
  A/RConn1 -- TPDL - Three-Phase Dynamic Load/LConn1
  TPDL - Three-Phase Dynamic Load/LConn2 -- B/RConn1
  C/RConn1 -- TPDL - Three-Phase Dynamic Load/LConn3
  n/RConn1 -- TPDL - Three-Phase Dynamic Load/LConn4

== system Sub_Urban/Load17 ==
  TPDL - Three-Phase Dynamic Load : myLibrary/TPDL - Three-Phase Dynamic Load  Load_Profile=LC(17)
  A : PMIOPort  Side=Left
  B : PMIOPort  Port=2  Side=Left
  C : PMIOPort  Port=3  Side=Left
  n : PMIOPort  Port=4  Side=Left
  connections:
  A/RConn1 -- TPDL - Three-Phase Dynamic Load/LConn1
  TPDL - Three-Phase Dynamic Load/LConn2 -- B/RConn1
  C/RConn1 -- TPDL - Three-Phase Dynamic Load/LConn3
  n/RConn1 -- TPDL - Three-Phase Dynamic Load/LConn4

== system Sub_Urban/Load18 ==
  SPDL - Single Phase Dynamic Load (Phasor) : myLibrary/SPDL - Single Phase Dynamic Load (Phasor)  Load_Profile=LC(18)  Phase=3
  Ph : PMIOPort  Side=Left
  n : PMIOPort  Port=2  Side=Left
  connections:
  Ph/RConn1 -- SPDL - Single Phase Dynamic Load (Phasor)/LConn1
  n/RConn1 -- SPDL - Single Phase Dynamic Load (Phasor)/LConn2

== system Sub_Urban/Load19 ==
  SPDL - Single Phase Dynamic Load (Phasor) : myLibrary/SPDL - Single Phase Dynamic Load (Phasor)  Load_Profile=LC(19)  Phase=2
  Ph : PMIOPort  Side=Left
  n : PMIOPort  Port=2  Side=Left
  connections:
  Ph/RConn1 -- SPDL - Single Phase Dynamic Load (Phasor)/LConn1
  n/RConn1 -- SPDL - Single Phase Dynamic Load (Phasor)/LConn2

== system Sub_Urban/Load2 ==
  TPDL - Three-Phase Dynamic Load : myLibrary/TPDL - Three-Phase Dynamic Load  Load_Profile=LC(2)
  A : PMIOPort  Side=Left
  B : PMIOPort  Port=2  Side=Left
  C : PMIOPort  Port=3  Side=Left
  n : PMIOPort  Port=4  Side=Left
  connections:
  A/RConn1 -- TPDL - Three-Phase Dynamic Load/LConn1
  TPDL - Three-Phase Dynamic Load/LConn2 -- B/RConn1
  C/RConn1 -- TPDL - Three-Phase Dynamic Load/LConn3
  n/RConn1 -- TPDL - Three-Phase Dynamic Load/LConn4

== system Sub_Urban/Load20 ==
  SPDL - Single Phase Dynamic Load (Phasor) : myLibrary/SPDL - Single Phase Dynamic Load (Phasor)  Load_Profile=LC(20)  Phase=2
  Ph : PMIOPort  Side=Left
  n : PMIOPort  Port=2  Side=Left
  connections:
  Ph/RConn1 -- SPDL - Single Phase Dynamic Load (Phasor)/LConn1
  n/RConn1 -- SPDL - Single Phase Dynamic Load (Phasor)/LConn2

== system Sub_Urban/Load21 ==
  SPDL - Single Phase Dynamic Load (Phasor) : myLibrary/SPDL - Single Phase Dynamic Load (Phasor)  Load_Profile=LC(21)  Phase=2
  Ph : PMIOPort  Side=Left
  n : PMIOPort  Port=2  Side=Left
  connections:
  Ph/RConn1 -- SPDL - Single Phase Dynamic Load (Phasor)/LConn1
  n/RConn1 -- SPDL - Single Phase Dynamic Load (Phasor)/LConn2

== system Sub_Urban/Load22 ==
  SPDL - Single Phase Dynamic Load (Phasor) : myLibrary/SPDL - Single Phase Dynamic Load (Phasor)  Load_Profile=LC(22)  Phase=1
  Ph : PMIOPort  Side=Left
  n : PMIOPort  Port=2  Side=Left
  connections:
  Ph/RConn1 -- SPDL - Single Phase Dynamic Load (Phasor)/LConn1
  n/RConn1 -- SPDL - Single Phase Dynamic Load (Phasor)/LConn2

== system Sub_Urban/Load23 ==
  SPDL - Single Phase Dynamic Load (Phasor) : myLibrary/SPDL - Single Phase Dynamic Load (Phasor)  Load_Profile=LC(23)  Phase=3
  Ph : PMIOPort  Side=Left
  n : PMIOPort  Port=2  Side=Left
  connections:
  Ph/RConn1 -- SPDL - Single Phase Dynamic Load (Phasor)/LConn1
  n/RConn1 -- SPDL - Single Phase Dynamic Load (Phasor)/LConn2

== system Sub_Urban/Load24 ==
  SPDL - Single Phase Dynamic Load (Phasor) : myLibrary/SPDL - Single Phase Dynamic Load (Phasor)  Load_Profile=LC(24)  Phase=1
  Ph : PMIOPort  Side=Left
  n : PMIOPort  Port=2  Side=Left
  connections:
  Ph/RConn1 -- SPDL - Single Phase Dynamic Load (Phasor)/LConn1
  n/RConn1 -- SPDL - Single Phase Dynamic Load (Phasor)/LConn2

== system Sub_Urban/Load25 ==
  SPDL - Single Phase Dynamic Load (Phasor) : myLibrary/SPDL - Single Phase Dynamic Load (Phasor)  Load_Profile=LC(25)  Phase=3
  Ph : PMIOPort  Side=Left
  n : PMIOPort  Port=2  Side=Left
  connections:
  Ph/RConn1 -- SPDL - Single Phase Dynamic Load (Phasor)/LConn1
  n/RConn1 -- SPDL - Single Phase Dynamic Load (Phasor)/LConn2

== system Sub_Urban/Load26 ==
  TPDL - Three-Phase Dynamic Load : myLibrary/TPDL - Three-Phase Dynamic Load  Load_Profile=LC(26)
  A : PMIOPort  Side=Left
  B : PMIOPort  Port=2  Side=Left
  C : PMIOPort  Port=3  Side=Left
  n : PMIOPort  Port=4  Side=Left
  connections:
  A/RConn1 -- TPDL - Three-Phase Dynamic Load/LConn1
  TPDL - Three-Phase Dynamic Load/LConn2 -- B/RConn1
  C/RConn1 -- TPDL - Three-Phase Dynamic Load/LConn3
  n/RConn1 -- TPDL - Three-Phase Dynamic Load/LConn4

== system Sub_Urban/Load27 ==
  SPDL - Single Phase Dynamic Load (Phasor) : myLibrary/SPDL - Single Phase Dynamic Load (Phasor)  Load_Profile=LC(27)  Phase=3
  Ph : PMIOPort  Side=Left
  n : PMIOPort  Port=2  Side=Left
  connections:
  Ph/RConn1 -- SPDL - Single Phase Dynamic Load (Phasor)/LConn1
  n/RConn1 -- SPDL - Single Phase Dynamic Load (Phasor)/LConn2

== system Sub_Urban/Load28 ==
  SPDL - Single Phase Dynamic Load (Phasor) : myLibrary/SPDL - Single Phase Dynamic Load (Phasor)  Load_Profile=LC(28)  Phase=2
  Ph : PMIOPort  Side=Left
  n : PMIOPort  Port=2  Side=Left
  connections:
  Ph/RConn1 -- SPDL - Single Phase Dynamic Load (Phasor)/LConn1
  n/RConn1 -- SPDL - Single Phase Dynamic Load (Phasor)/LConn2

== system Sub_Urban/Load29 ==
  TPDL - Three-Phase Dynamic Load : myLibrary/TPDL - Three-Phase Dynamic Load  Load_Profile=LC(29)
  A : PMIOPort  Side=Left
  B : PMIOPort  Port=2  Side=Left
  C : PMIOPort  Port=3  Side=Left
  n : PMIOPort  Port=4  Side=Left
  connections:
  A/RConn1 -- TPDL - Three-Phase Dynamic Load/LConn1
  TPDL - Three-Phase Dynamic Load/LConn2 -- B/RConn1
  C/RConn1 -- TPDL - Three-Phase Dynamic Load/LConn3
  n/RConn1 -- TPDL - Three-Phase Dynamic Load/LConn4

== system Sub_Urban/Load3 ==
  SPDL - Single Phase Dynamic Load (Phasor) : myLibrary/SPDL - Single Phase Dynamic Load (Phasor)  Load_Profile=LC(3)  Phase=1
  Ph : PMIOPort  Side=Left
  n : PMIOPort  Port=2  Side=Left
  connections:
  Ph/RConn1 -- SPDL - Single Phase Dynamic Load (Phasor)/LConn1
  n/RConn1 -- SPDL - Single Phase Dynamic Load (Phasor)/LConn2

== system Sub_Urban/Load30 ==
  SPDL - Single Phase Dynamic Load (Phasor) : myLibrary/SPDL - Single Phase Dynamic Load (Phasor)  Load_Profile=LC(30)  Phase=3
  Ph : PMIOPort  Side=Left
  n : PMIOPort  Port=2  Side=Left
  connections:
  Ph/RConn1 -- SPDL - Single Phase Dynamic Load (Phasor)/LConn1
  n/RConn1 -- SPDL - Single Phase Dynamic Load (Phasor)/LConn2

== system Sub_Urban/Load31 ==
  SPDL - Single Phase Dynamic Load (Phasor) : myLibrary/SPDL - Single Phase Dynamic Load (Phasor)  Load_Profile=LC(31)  Phase=2
  Ph : PMIOPort  Side=Left
  n : PMIOPort  Port=2  Side=Left
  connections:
  Ph/RConn1 -- SPDL - Single Phase Dynamic Load (Phasor)/LConn1
  n/RConn1 -- SPDL - Single Phase Dynamic Load (Phasor)/LConn2

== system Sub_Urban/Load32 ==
  TPDL - Three-Phase Dynamic Load : myLibrary/TPDL - Three-Phase Dynamic Load  Load_Profile=LC(32)
  A : PMIOPort  Side=Left
  B : PMIOPort  Port=2  Side=Left
  C : PMIOPort  Port=3  Side=Left
  n : PMIOPort  Port=4  Side=Left
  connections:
  A/RConn1 -- TPDL - Three-Phase Dynamic Load/LConn1
  TPDL - Three-Phase Dynamic Load/LConn2 -- B/RConn1
  C/RConn1 -- TPDL - Three-Phase Dynamic Load/LConn3
  n/RConn1 -- TPDL - Three-Phase Dynamic Load/LConn4

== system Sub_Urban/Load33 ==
  SPDL - Single Phase Dynamic Load (Phasor) : myLibrary/SPDL - Single Phase Dynamic Load (Phasor)  Load_Profile=LC(33)  Phase=1
  Ph : PMIOPort  Side=Left
  n : PMIOPort  Port=2  Side=Left
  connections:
  Ph/RConn1 -- SPDL - Single Phase Dynamic Load (Phasor)/LConn1
  n/RConn1 -- SPDL - Single Phase Dynamic Load (Phasor)/LConn2

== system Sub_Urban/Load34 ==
  SPDL - Single Phase Dynamic Load (Phasor) : myLibrary/SPDL - Single Phase Dynamic Load (Phasor)  Load_Profile=LC(34)  Phase=3
  Ph : PMIOPort  Side=Left
  n : PMIOPort  Port=2  Side=Left
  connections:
  Ph/RConn1 -- SPDL - Single Phase Dynamic Load (Phasor)/LConn1
  n/RConn1 -- SPDL - Single Phase Dynamic Load (Phasor)/LConn2

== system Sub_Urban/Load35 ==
  SPDL - Single Phase Dynamic Load (Phasor) : myLibrary/SPDL - Single Phase Dynamic Load (Phasor)  Load_Profile=LC(35)  Phase=1
  Ph : PMIOPort  Side=Left
  n : PMIOPort  Port=2  Side=Left
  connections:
  Ph/RConn1 -- SPDL - Single Phase Dynamic Load (Phasor)/LConn1
  n/RConn1 -- SPDL - Single Phase Dynamic Load (Phasor)/LConn2

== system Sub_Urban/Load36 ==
  SPDL - Single Phase Dynamic Load (Phasor) : myLibrary/SPDL - Single Phase Dynamic Load (Phasor)  Load_Profile=LC(36)  Phase=3
  Ph : PMIOPort  Side=Left
  n : PMIOPort  Port=2  Side=Left
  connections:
  Ph/RConn1 -- SPDL - Single Phase Dynamic Load (Phasor)/LConn1
  n/RConn1 -- SPDL - Single Phase Dynamic Load (Phasor)/LConn2

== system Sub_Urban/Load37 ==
  SPDL - Single Phase Dynamic Load (Phasor) : myLibrary/SPDL - Single Phase Dynamic Load (Phasor)  Load_Profile=LC(37)  Phase=3
  Ph : PMIOPort  Side=Left
  n : PMIOPort  Port=2  Side=Left
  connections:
  Ph/RConn1 -- SPDL - Single Phase Dynamic Load (Phasor)/LConn1
  n/RConn1 -- SPDL - Single Phase Dynamic Load (Phasor)/LConn2

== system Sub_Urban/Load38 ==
  SPDL - Single Phase Dynamic Load (Phasor) : myLibrary/SPDL - Single Phase Dynamic Load (Phasor)  Load_Profile=LC(38)  Phase=2
  Ph : PMIOPort  Side=Left
  n : PMIOPort  Port=2  Side=Left
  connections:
  Ph/RConn1 -- SPDL - Single Phase Dynamic Load (Phasor)/LConn1
  n/RConn1 -- SPDL - Single Phase Dynamic Load (Phasor)/LConn2

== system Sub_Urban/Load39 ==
  SPDL - Single Phase Dynamic Load (Phasor) : myLibrary/SPDL - Single Phase Dynamic Load (Phasor)  Load_Profile=LC(39)  Phase=1
  Ph : PMIOPort  Side=Left
  n : PMIOPort  Port=2  Side=Left
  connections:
  Ph/RConn1 -- SPDL - Single Phase Dynamic Load (Phasor)/LConn1
  n/RConn1 -- SPDL - Single Phase Dynamic Load (Phasor)/LConn2

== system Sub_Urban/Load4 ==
  SPDL - Single Phase Dynamic Load (Phasor) : myLibrary/SPDL - Single Phase Dynamic Load (Phasor)  Load_Profile=LC(4)  Phase=3
  Ph : PMIOPort  Side=Left
  n : PMIOPort  Port=2  Side=Left
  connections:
  Ph/RConn1 -- SPDL - Single Phase Dynamic Load (Phasor)/LConn1
  n/RConn1 -- SPDL - Single Phase Dynamic Load (Phasor)/LConn2

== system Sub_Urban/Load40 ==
  SPDL - Single Phase Dynamic Load (Phasor) : myLibrary/SPDL - Single Phase Dynamic Load (Phasor)  Load_Profile=LC(7)  Phase=2
  Ph : PMIOPort  Side=Left
  n : PMIOPort  Port=2  Side=Left
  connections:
  Ph/RConn1 -- SPDL - Single Phase Dynamic Load (Phasor)/LConn1
  n/RConn1 -- SPDL - Single Phase Dynamic Load (Phasor)/LConn2

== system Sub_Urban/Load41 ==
  TPDL - Three-Phase Dynamic Load : myLibrary/TPDL - Three-Phase Dynamic Load  Load_Profile=LC(41)
  A : PMIOPort  Side=Left
  B : PMIOPort  Port=2  Side=Left
  C : PMIOPort  Port=3  Side=Left
  n : PMIOPort  Port=4  Side=Left
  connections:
  A/RConn1 -- TPDL - Three-Phase Dynamic Load/LConn1
  TPDL - Three-Phase Dynamic Load/LConn2 -- B/RConn1
  C/RConn1 -- TPDL - Three-Phase Dynamic Load/LConn3
  n/RConn1 -- TPDL - Three-Phase Dynamic Load/LConn4

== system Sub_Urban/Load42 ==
  SPDL - Single Phase Dynamic Load (Phasor) : myLibrary/SPDL - Single Phase Dynamic Load (Phasor)  Load_Profile=LC(42)  Phase=3
  Ph : PMIOPort  Side=Left
  n : PMIOPort  Port=2  Side=Left
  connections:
  Ph/RConn1 -- SPDL - Single Phase Dynamic Load (Phasor)/LConn1
  n/RConn1 -- SPDL - Single Phase Dynamic Load (Phasor)/LConn2
